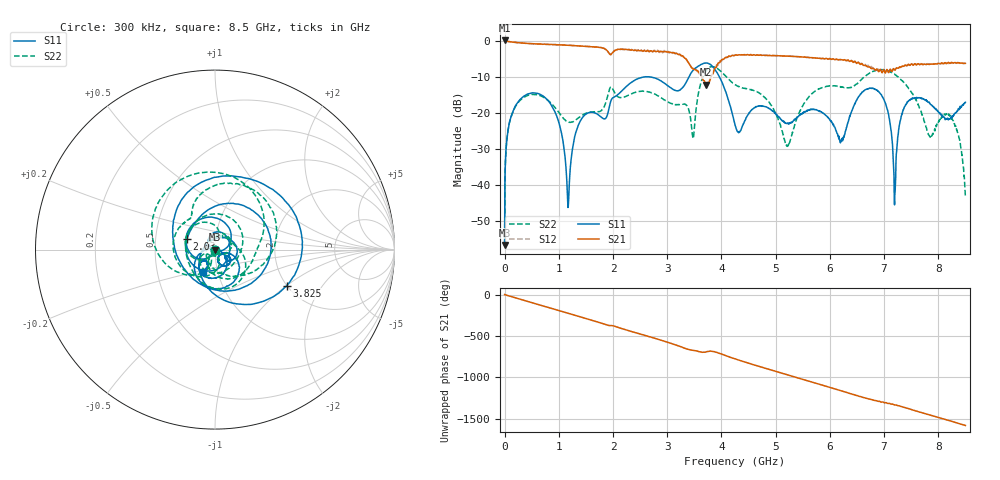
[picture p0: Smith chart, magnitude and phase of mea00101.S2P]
!Agilent Technologies,E5071B,MY42402595,A.08.01
!Date: Tue Jan 02 10:12:30 2001
!Data & Calibration Information:
!Freq	S11:SOLT2(ON)	S21:SOLT2(ON)	S12:SOLT2(ON)	S22:SOLT2(ON)
# Hz S dB R 50
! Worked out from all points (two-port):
!   1601 points, 300 kHz to 8.5 GHz, reference 50 ohm
!   highest |S21| = 0.04 dB at 300 kHz (marker M1); lowest = -12.2 dB at 3.719 GHz (marker M2)
!   |S21| within 3 dB of the highest: start of sweep to 1.902 GHz; 2.014 GHz to 2.601 GHz (586.6 MHz wide, 25.4 % of centre)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
!   lowest |S11| = -56.6 dB at 300 kHz (marker M3), VSWR 1.00, Z = 50.1 - j0.047 ohm
!   |S11| at or under -10 dB: start of sweep to 2.64 GHz; 2.658 GHz to 3.403 GHz (744.3 MHz wide, 24.6 % of centre); 3.961 GHz to end of sweep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
!   |S22| runs from -57.0 to -7.2 dB; largest |S21 - S12| = 0.032
!   S11 on the Smith chart (normalised r, x): 300 kHz: 1.00, -0.00; 2.03 GHz: 0.73, +0.09; 3.825 GHz: 1.99, -1.00; 8.5 GHz: 0.85, -0.21
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300000  -56.64 -18.6  0.04 0.1  -0.01 -0.1  -56.96 -130.5
1.809186e8  -18.69 -157.4  -0.49 -37.0  -0.47 -37.0  -18.78 -151.7
8.555823e8  -17.74 47.6  -1.06 -165.2  -1.08 -165.1  -17.30 91.4
1.169009e9  -46.25 -96.7  -1.28 134.5  -1.28 134.6  -22.54 78.3
1.418687e9  -21.71 109.3  -1.54 86.7  -1.53 86.7  -20.83 75.6
2.029603e9  -15.58 159.7  -2.73 -22.8  -2.86 -22.5  -14.40 -116.6
2.374904e9  -11.20 69.4  -2.68 -93.1  -2.78 -92.0  -14.54 125.3
2.837075e9  -10.77 -30.3  -2.97 178.4  -2.92 176.3  -15.37 25.3
3.474552e9  -8.29 99.6  -7.84 47.1  -7.65 46.9  -27.02 -138.7
3.718919e9  -6.21 10.8  -12.19 28.5  -11.76 28.3  -8.32 155.7
3.825165e9  -6.99 -26.9  -9.48 33.9  -9.86 36.6  -7.22 108.0
4.25015e9  -23.33 -179.9  -4.03 -55.5  -4.05 -55.8  -12.21 5.7
4.871691e9  -18.78 -28.4  -4.15 178.3  -4.12 178.0  -16.92 -89.8
5.222303e9  -22.85 -33.7  -4.31 109.9  -4.30 109.6  -29.12 -94.8
5.668537e9  -19.14 -45.8  -4.73 23.4  -4.78 23.3  -14.72 -126.8
6.242267e9  -27.00 -32.8  -5.44 -87.6  -5.34 -87.6  -12.92 135.8
7.086925e9  -20.74 -164.0  -8.87 126.4  -8.43 123.6  -8.51 27.6
7.198483e9  -42.56 50.0  -8.19 108.3  -7.99 107.9  -9.40 7.0
7.384414e9  -18.24 -60.2  -6.78 75.7  -6.94 74.7  -11.96 -27.2
7.782838e9  -16.52 -124.3  -6.57 -2.6  -6.60 -2.3  -24.19 -141.2
8.234384e9  -21.21 -120.0  -6.12 -87.4  -6.15 -88.9  -21.08 4.2
8.5e9  -17.10 -118.2  -6.31 -140.3  -6.30 -141.1  -43.27 -123.6
